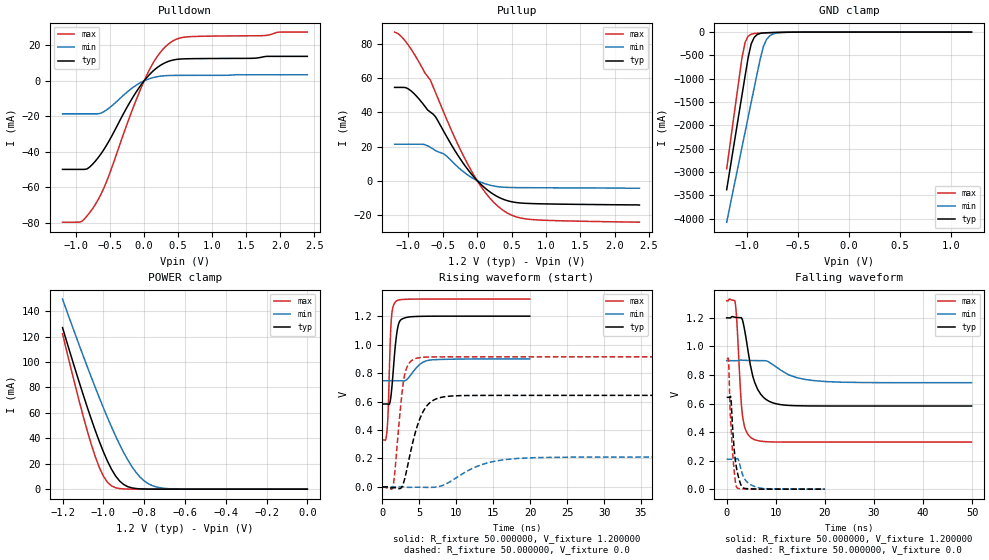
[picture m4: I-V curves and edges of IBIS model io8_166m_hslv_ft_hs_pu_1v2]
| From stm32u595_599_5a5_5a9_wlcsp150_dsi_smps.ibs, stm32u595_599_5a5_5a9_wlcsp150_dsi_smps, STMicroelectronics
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|   Model io8_166m_hslv_ft_hs_pu_1v2
[Model]  io8_166m_hslv_ft_hs_pu_1v2
Model_type I/O
Polarity   Non-Inverting
Enable   Active-Low
Vinl =   0.360000V
Vinh =   0.840000V
Vmeas =  0.600000V
Cref =   50.000000pF
Rref =   100.000000M
Vref =   0.0V
C_comp   3.151700pF   3.087200pF   3.197900pF
[Temperature Range]   25.000000   0.140000k   -40.000000
[Pullup Reference]   1.200000V   0.900000V   1.320000V
[Pulldown Reference]   0.0V   0.0V   0.0V
[POWER Clamp Reference]   1.200000V   0.900000V   1.320000V
[GND Clamp Reference]   0.0V   0.0V   0.0V
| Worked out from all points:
|   slope of the pulldown table from 0 to 0.18 V, typ, clamps not added: 25.4 ohm
|   slope of the pullup table from 0 to 0.18 V, typ, clamps not added: 27.8 ohm
|   GND clamp passes 1 mA (typ) near -0.51 V on its own axis
|   POWER clamp passes 1 mA (typ) near -0.86 V on its own axis
|   rising waveform, R_fixture 50.000000, V_fixture 1.200000: 20-80 % time 647ps typ, 1.58ns min, 369ps max; typ from 0.583 V to 1.2 V
|   rising waveform, R_fixture 50.000000, V_fixture 0.0: 20-80 % time 2.04ns typ, 4.82ns min, 1.01ns max; typ from 0 V to 0.643 V
|   falling waveform, R_fixture 50.000000, V_fixture 1.200000: 20-80 % time 2.37ns typ, 5.33ns min, 1.03ns max; typ from 1.2 V to 0.583 V
|   falling waveform, R_fixture 50.000000, V_fixture 0.0: 20-80 % time 1.04ns typ, 1.74ns min, 829ps max; typ from 0.643 V to 0 V
[Pulldown]
|Voltage   I(typ)   I(min)   I(max)
-1.2V     -49.86mA   -18.57mA   -79.56mA
-920mV    -49.86mA   -18.57mA   -79.19mA
-840mV    -49.6mA    -18.57mA   -76.08mA
-720mV    -45.32mA   -18.57mA   -69.74mA
-560mV    -36.71mA   -16.58mA   -57.44mA
-200mV    -11.43mA   -4.74mA    -19.03mA
0V        0A         0A         0A
160mV     6.477mA    2.075mA    11.78mA
360mV     10.99mA    2.99mA     20.81mA
480mV     12.07mA    3.054mA    23.52mA
640mV     12.43mA    3.075mA    24.76mA
2.4V      13.77mA    3.425mA    27.43mA
[Pullup]
|Voltage   I(typ)   I(min)   I(max)
-1.2V     54.73mA    21.36mA    87.24mA
-1.04V    54.63mA    21.36mA    81.75mA
-880mV    49.53mA    21.36mA    72.03mA
-680mV    40.22mA    19.54mA    59.02mA
-600mV    37.17mA    17.44mA    51.23mA
-480mV    28.49mA    15.58mA    39.53mA
-80mV     3.667mA    1.75mA     5.47mA
120mV     -4.592mA   -1.936mA   -7.077mA
360mV     -10.68mA   -3.85mA    -16.99mA
560mV     -12.87mA   -4.135mA   -21.24mA
760mV     -13.48mA   -4.204mA   -22.78mA
2.36V     -14.4mA    -4.5mA     -24.47mA
[GND_clamp]
|Voltage   I(typ)   I(min)   I(max)
-1.2V     -3.379A    -4.076A    -2.932A
-1.05V    -1.35A     -2.47A     -550.7mA
-1.02V    -947.8mA   -2.149A    -221.5mA
-990mV    -552.4mA   -1.829A    -88.44mA
-960mV    -255.3mA   -1.51A     -44.87mA
-930mV    -111.8mA   -1.191A    -30.68mA
-870mV    -28.36mA   -564.6mA   -21.34mA
-840mV    -18.65mA   -309.5mA   -18.49mA
-810mV    -14.07mA   -161.6mA   -15.92mA
-780mV    -11.37mA   -83.33mA   -13.53mA
-600mV    -3.009mA   -4.322mA   -3.091mA
1.2V      0A         13.65nA    0A
[POWER_clamp]
|Voltage   I(typ)   I(min)   I(max)
-1.2V     127mA      149.4mA    122.2mA
-1.12V    84.98mA    114mA      70.29mA
-1.06V    55.52mA    88.42mA    35.69mA
-1.02V    37.64mA    72.04mA    17.19mA
-1V       29.52mA    64.13mA    10.33mA
-960mV    15.7mA     48.99mA    2.596mA
-900mV    3.636mA    28.77mA    207.8uA
-840mV    502.9uA    13.24mA    43.19uA
-800mV    129uA      6.535mA    43.19uA
-740mV    26.51uA    1.726mA    43.19uA
-620mV    25.02uA    82.33uA    35.3uA
0V        0A         17.36nA    0A
[Ramp]
| variable   typ   min   max
dV/dt_r  0.38569/2.03993n   0.12564/4.81368n   0.54818/1.00416n
dV/dt_f  0.37043/2.36888n   92.35800m/5.31956n  0.59405/1.02308n
R_load = 50.000000
[Rising Waveform]
R_fixture= 50.000000
V_fixture= 1.200000
V_fixture_min= 0.900000
V_fixture_max= 1.320000
|time   V(typ)   V(min)   V(max)
0s        582.7mV    746.1mV    330.1mV
600.6ps   583mV      746.1mV    380.8mV
800.8ps   581mV      746.1mV    554.2mV
1.041ns   596.7mV    746.1mV    983.9mV
1.201ns   655.4mV    746.1mV    1.169V
1.842ns   1.036V     746.2mV    1.304V
2.322ns   1.162V     746.2mV    1.315V
3.483ns   1.193V     763.8mV    1.319V
6.527ns   1.2V       892.4mV    1.32V
19.94ns   1.2V       900mV      1.32V
[Rising Waveform]
R_fixture= 50.000000
V_fixture= 0.0
V_fixture_min= 0.0
V_fixture_max= 0.0
|time   V(typ)   V(min)   V(max)
0s        427.2uV    495.3uV    343.3uV
1.401ns   -5.82mV    476.2uV    -6.76mV
2.903ns   35.19mV    -13.79uV   756.2mV
3.504ns   169.7mV    -2.699mV   860mV
4.505ns   390.6mV    -1.802mV   901.9mV
6.206ns   581.1mV    -3.179mV   913mV
8.909ns   636.9mV    29.47mV    914mV
13.41ns   643.1mV    156.3mV    914.1mV
18.22ns   643.3mV    200.1mV    914.1mV
49.85ns   643.4mV    210mV      914.2mV
[Falling Waveform]
R_fixture= 50.000000
V_fixture= 1.200000
V_fixture_min= 0.900000
V_fixture_max= 1.320000
|time   V(typ)   V(min)   V(max)
0s        1.2V       900mV      1.32V
1.702ns   1.204V     899.9mV    1.315V
2.002ns   1.203V     899.6mV    1.207V
3.203ns   1.187V     903.2mV    520.6mV
3.904ns   1.065V     902.1mV    412mV
5.305ns   792.4mV    900.9mV    353.4mV
7.508ns   643mV      900.3mV    334.2mV
11.01ns   592.2mV    833.4mV    330.4mV
20.02ns   582.8mV    754.1mV    330.1mV
49.85ns   582.7mV    746.1mV    330.1mV
[Falling Waveform]
R_fixture= 50.000000
V_fixture= 0.0
V_fixture_min= 0.0
V_fixture_max= 0.0
|time   V(typ)   V(min)   V(max)
0s        643.4mV    210mV      914.2mV
400.4ps   643.4mV    210mV      885.7mV
680.7ps   647.8mV    210.1mV    574.2mV
840.8ps   642.7mV    210.1mV    464.2mV
1.161ns   457.1mV    210.1mV    275.2mV
1.481ns   298.6mV    209.9mV    144.6mV
2.082ns   133.9mV    214mV      11.7mV
3.203ns   13.66mV    105.8mV    2.096mV
5.646ns   1.556mV    19.55mV    527.9uV
19.94ns   427.2uV    495.3uV    343.3uV
